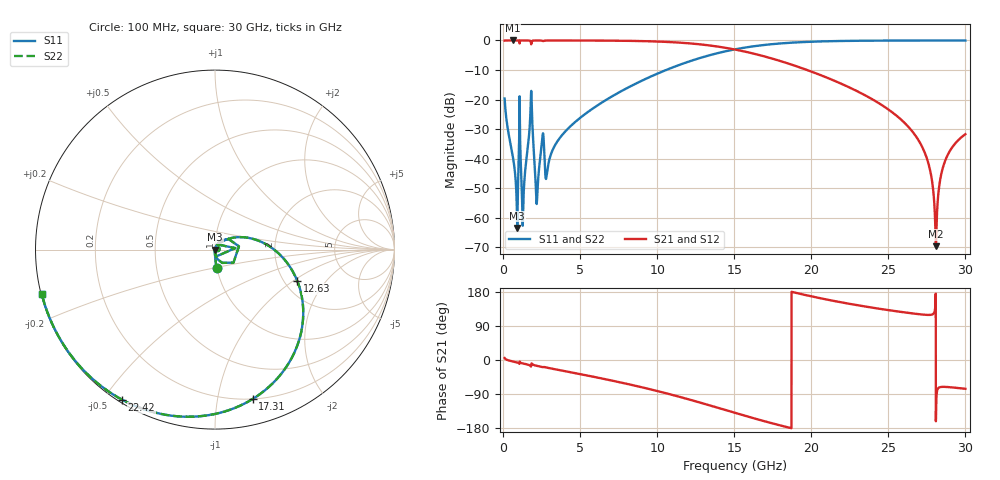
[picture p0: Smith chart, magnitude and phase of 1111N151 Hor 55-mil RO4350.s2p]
# GHz S MA R 50
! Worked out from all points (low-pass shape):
!   3201 points, 100 MHz to 30 GHz, reference 50 ohm
!   highest |S21| = 0.00 dB at 613.9 MHz (marker M1); lowest = -69.7 dB at 28.08 GHz (marker M2)
!   |S21| within 3 dB of the highest: start of sweep to 14.98 GHz
!   lowest |S11| = -63.5 dB at 922.2 MHz (marker M3), VSWR 1.00, Z = 50.1 + j0.00816 ohm
!   |S11| at or under -10 dB: start of sweep to 10.58 GHz
!   |S22| runs from -63.5 to 0.0 dB; largest |S21 - S12| = 0
!   S11 on the Smith chart (normalised r, x): 100 MHz: 1.00, -0.21; 12.63 GHz: 2.34, -1.08; 17.31 GHz: 0.20, -1.27; 22.42 GHz: 0.01, -0.56; 30 GHz: 0.00, -0.13
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0.1  0.104 -84.6  0.9943 5.3  0.9943 5.3  0.104 -84.6
0.6139062  0.01155 -91.6  0.9994 -3.7  0.9994 -3.7  0.01155 -91.6
0.92225  0.0006706 7.0  0.9992 -6.5  0.9992 -6.5  0.0006706 7.0
1.099781  0.02582 -84.3  0.9942 -6.3  0.9942 -6.3  0.02582 -84.3
1.352062  0.003126 66.7  0.9991 -9.7  0.9991 -9.7  0.003126 66.7
1.791219  0.08003 45.8  0.9603 -16.6  0.9603 -16.6  0.08003 45.8
2.202344  0.001971 17.1  0.9981 -15.5  0.9981 -15.5  0.001971 17.1
2.529375  0.02009 43.2  0.9901 -18.7  0.9901 -18.7  0.02009 43.2
2.856406  0.005916 44.2  0.9971 -20.3  0.9971 -20.3  0.005916 44.2
5.089563  0.05098 50.8  0.997 -37.9  0.997 -37.9  0.05098 50.8
10.06978  0.2781 7.1  0.9574 -82.5  0.9574 -82.5  0.2781 7.1
12.62997  0.4909 -20.9  0.8668 -110.6  0.8668 -110.6  0.4909 -20.9
15.05  0.7068 -49.8  0.7015 -139.5  0.7015 -139.5  0.7068 -49.8
17.31119  0.8579 -75.8  0.506 -165.5  0.506 -165.5  0.8579 -75.8
20.03956  0.9519 -102.6  0.2947 167.7  0.2947 167.7  0.9519 -102.6
22.42222  0.9834 -121.7  0.1624 148.6  0.1624 148.6  0.9834 -121.7
25.01978  0.9946 -139.0  0.0673 131.5  0.0673 131.5  0.9946 -139.0
27.27163  0.9968 -151.9  0.0143 119.7  0.0143 119.7  0.9968 -151.9
27.73881  0.9969 -154.3  0.005838 119.2  0.005838 119.2  0.9969 -154.3
28.08453  0.9969 -156.1  0.0003288 -161.6  0.0003288 -161.6  0.9969 -156.1
28.68253  0.9969 -159.2  0.00913 -70.9  0.00913 -70.9  0.9969 -159.2
30  0.9965 -165.6  0.02588 -76.0  0.02588 -76.0  0.9965 -165.6
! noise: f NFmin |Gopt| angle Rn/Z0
0.1  0.0006461  0.7275  1.011  0.0004715
3.417  0.00898  0.4466  23.44  0.002607
6.743  0.01403  0.363  42.53  0.0031
10.06  0.02123  0.3914  58.22  0.004518
13.39  0.03207  0.4771  73.21  0.007187
16.7  0.05152  0.6101  90.39  0.01289
20.03  0.09412  0.7602  110.1  0.02709
23.35  0.2158  0.887  130.2  0.07493
26.67  1.006  0.9741  148.8  0.6437
30  1.048  0.9742  165.5  0.151
